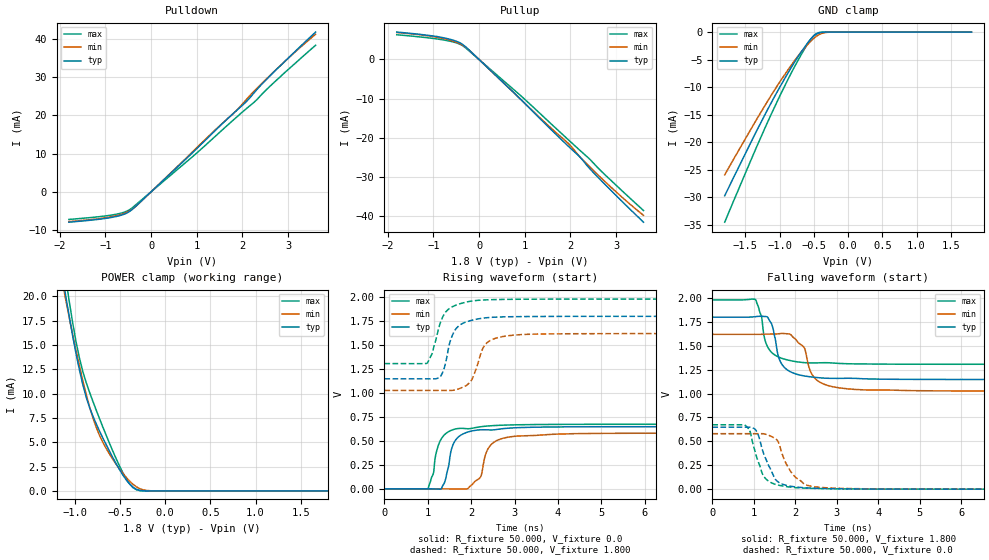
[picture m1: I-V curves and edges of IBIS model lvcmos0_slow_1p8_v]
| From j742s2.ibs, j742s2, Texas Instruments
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|   slow_1p8_v
[Model]   lvcmos0_slow_1p8_v
Model_type I/O
Polarity   Non-Inverting
Enable   Active-High
Vinl = 0
Vinh = 0.8
Vmeas = 0.9
Vref = 1.8
Cref = 2pF
Rref = 100000
|   typ   min   max
C_comp   2.800pF   2.558pF   3.038pF
[Voltage Range]   1.8   1.62   1.98
[Temperature Range]   27   150   -40
[Pullup Reference]   1.8   1.62   1.98
[Pulldown Reference]   0   0   0
[Power Clamp Reference]   1.8   1.62   1.98
[GND Clamp Reference]   0   0   0
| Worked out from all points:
|   slope of the pulldown table from 0 to 0.27 V, typ, clamps not added: 88.7 ohm
|   slope of the pullup table from 0 to 0.27 V, typ, clamps not added: 89.7 ohm
|   GND clamp passes 1 mA (typ) near -0.52 V on its own axis
|   POWER clamp passes 1 mA (typ) near -0.42 V on its own axis
|   rising waveform, R_fixture 50.000, V_fixture 0.0: 20-80 % time 234ps typ, 265ps min, 232ps max; typ from 0 V to 0.648 V
|   rising waveform, R_fixture 50.000, V_fixture 1.800: 20-80 % time 260ps typ, 296ps min, 294ps max; typ from 1.15 V to 1.8 V
|   falling waveform, R_fixture 50.000, V_fixture 1.800: 20-80 % time 258ps typ, 334ps min, 257ps max; typ from 1.8 V to 1.15 V
|   falling waveform, R_fixture 50.000, V_fixture 0.0: 20-80 % time 343ps typ, 411ps min, 294ps max; typ from 0.648 V to 0 V
[Pulldown]
|Voltage   I(typ)   I(min)   I(max)
-1.8V     -7.963mA   -7.801mA   -7.241mA
-1.194V   -7.271mA   -7.118mA   -6.591mA
-808mV    -6.583mA   -6.398mA   -5.977mA
-588mV    -5.86mA    -5.668mA   -5.345mA
-422mV    -4.71mA    -4.654mA   -4.282mA
-257mV    -2.902mA   -2.957mA   -2.608mA
955mV     10.79mA    11.03mA    9.687mA
1.837V    20.92mA    20.94mA    19.19mA
2.057V    23.3mA     23.79mA    21.49mA
2.278V    26.26mA    26.63mA    23.71mA
2.773V    32.37mA    32.42mA    29.54mA
3.6V      41.82mA    41.24mA    38.38mA
[Pullup]
|Voltage   I(typ)   I(min)   I(max)
-1.8V     6.998mA    6.891mA    6.313mA
-918mV    5.872mA    5.673mA    5.243mA
-588mV    5.01mA     4.789mA    4.536mA
-367mV    3.923mA    3.703mA    3.583mA
-202mV    2.255mA    2.239mA    2.047mA
955mV     -10.69mA   -10.66mA   -9.684mA
1.506V    -17.07mA   -16.77mA   -15.65mA
1.947V    -22.06mA   -21.35mA   -20.42mA
2.222V    -25.07mA   -25.04mA   -23.35mA
2.443V    -28.13mA   -27.65mA   -25.69mA
2.773V    -32.1mA    -31.37mA   -29.62mA
3.6V      -41.55mA   -39.8mA    -38.57mA
[GND_clamp]
|Voltage   I(typ)   I(min)   I(max)
-1.8V     -29.72mA   -25.92mA   -34.52mA
-1.318V   -17.54mA   -15.51mA   -20.38mA
-1.132V   -13.09mA   -11.7mA    -15.22mA
-984mV    -9.729mA   -8.822mA   -11.3mA
-798mV    -5.797mA   -5.487mA   -6.696mA
-612mV    -2.352mA   -2.574mA   -2.564mA
-538mV    -1.174mA   -1.582mA   -1.166mA
-464mV    -368uA     -771.3uA   -275.5uA
-353mV    -15.75uA   -129.3uA   -4.378uA
-241mV    -383.4nA   -10.85uA   -119.1nA
1.8V      0A         0A         0A
[POWER_clamp]
|Voltage   I(typ)   I(min)   I(max)
-1.8V     63.47mA    56.87mA    71.37mA
-1.132V   21.93mA    21.29mA    24mA
-1.095V   19.85mA    19.49mA    21.65mA
-1.058V   17.84mA    17.74mA    19.39mA
-984mV    14.08mA    14.39mA    15.3mA
-909mV    10.9mA     11.31mA    12.25mA
-761mV    6.887mA    6.531mA    8.298mA
-649mV    4.716mA    4.334mA    5.678mA
-464mV    1.598mA    1.771mA    1.827mA
-315mV    160.7uA    409.8uA    112.2uA
-130mV    308nA      7.74uA     148.3nA
1.8V      0A         0A         0A
[Ramp]
| variable   typ   min   max
dV/dt_r   0.389/0.233n   0.348/0.263n   0.404/0.232n
dV/dt_f   0.391/0.258n   0.356/0.335n   0.404/0.256n
R_load = 50.000
[Rising Waveform]
R_fixture= 50.000
V_fixture= 0.0
|time   V(typ)   V(min)   V(max)
0s        961.2nV    20.53uV    1.691uV
1.003ns   104uV      18.77uV    172.7uV
1.297ns   -3.062mV   -5.319uV   510.4mV
1.411ns   101.2mV    76.52uV    574.7mV
1.555ns   427.3mV    -706.1uV   612.8mV
1.681ns   530.4mV    -1.883mV   628.3mV
2.212ns   615.3mV    120.5mV    647.4mV
2.457ns   614.4mV    459.8mV    657.9mV
2.91ns    634.3mV    543mV      666.5mV
10ns      648.3mV    580.6mV    673.9mV
[Rising Waveform]
R_fixture= 50.000
V_fixture= 1.800
V_fixture_min= 1.620
V_fixture_max= 1.980
|time   V(typ)   V(min)   V(max)
0s        1.148V     1.027V     1.307V
979ps     1.148V     1.027V     1.31V
1.103ns   1.147V     1.027V     1.414V
1.283ns   1.167V     1.027V     1.723V
1.416ns   1.327V     1.027V     1.847V
1.611ns   1.643V     1.03V      1.909V
2.026ns   1.76V      1.149V     1.96V
2.321ns   1.784V     1.503V     1.971V
2.844ns   1.795V     1.597V     1.977V
10ns      1.8V       1.62V      1.98V
[Falling Waveform]
R_fixture= 50.000
V_fixture= 1.800
V_fixture_min= 1.620
V_fixture_max= 1.980
|time   V(typ)   V(min)   V(max)
0s        1.8V       1.62V      1.98V
1.042ns   1.805V     1.62V      1.982V
1.323ns   1.803V     1.622V     1.496V
1.456ns   1.69V      1.623V     1.42V
1.648ns   1.326V     1.629V     1.373V
2.02ns    1.204V     1.561V     1.334V
2.214ns   1.185V     1.48V      1.324V
2.461ns   1.171V     1.165V     1.321V
3.059ns   1.159V     1.06V      1.315V
10ns      1.148V     1.027V     1.307V
[Falling Waveform]
R_fixture= 50.000
V_fixture= 0.0
V_fixture_min= 0.0
V_fixture_max= 0.0
|time   V(typ)   V(min)   V(max)
0s        648.3mV    580.6mV    673.9mV
775ps     648.3mV    580.6mV    671.8mV
905ps     648.5mV    580.6mV    607.9mV
1.017ns   631.4mV    580.6mV    412.8mV
1.281ns   323.2mV    575mV      111.3mV
1.571ns   79.82mV    507.1mV    44.39mV
1.759ns   42.72mV    283.3mV    28.53mV
2.204ns   15.58mV    57.04mV    11.36mV
2.608ns   7.835mV    18.53mV    6.216mV
10ns      47.85uV    118uV      30.83uV
